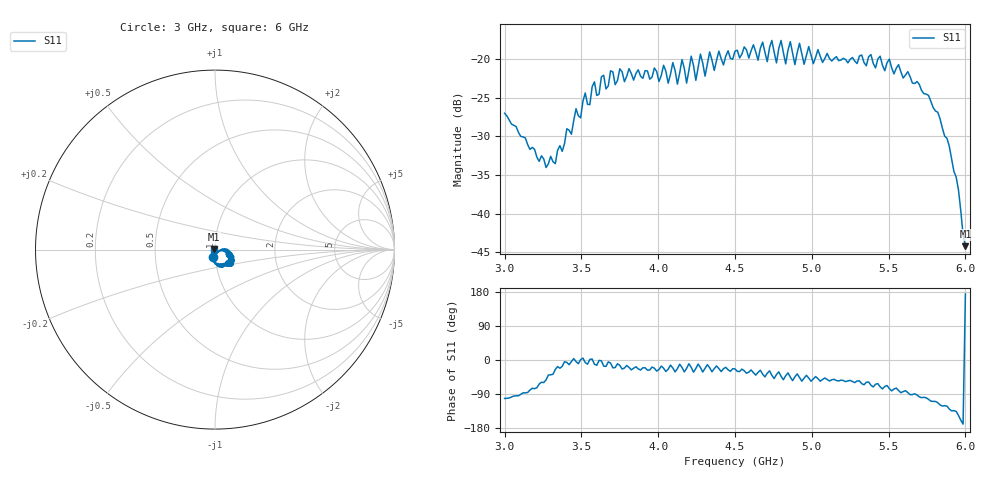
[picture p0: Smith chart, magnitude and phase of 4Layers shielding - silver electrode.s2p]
!  03/07/2025  16:02:48
! Ref Plane: 0.000 mm
# MHZ S MA R  50
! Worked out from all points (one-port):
!   201 points, 3 GHz to 6 GHz, reference 50 ohm
!   lowest |S11| = -44.2 dB at 6 GHz (marker M1), VSWR 1.01, Z = 49.4 + j0.0619 ohm
!   |S11| at or under -10 dB: start of sweep to end of sweep
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3000  0.0446 -101.5
3270  0.01987 -52.5
3375  0.02527 -16.7
3525  0.06031 -6.9
3555  0.0507 1.4
3585  0.0712 -11.3
3750  0.08648 -14.1
4005  0.07155 -25.4
4035  0.09118 -21.6
4065  0.06976 -24.2
4095  0.09481 -21.0
4125  0.06882 -22.9
4155  0.09917 -19.6
4185  0.06993 -22.0
4215  0.1044 -19.4
4245  0.07283 -22.4
4275  0.1077 -19.8
4305  0.07751 -22.3
4335  0.1112 -20.4
4365  0.08439 -22.8
4395  0.1125 -22.7
4500  0.1124 -23.6
4875  0.1088 -54.4
5250  0.09965 -53.9
5625  0.08282 -85.8
5880  0.0307 -121.7
5955  0.01422 -146.3
6000  0.006155 174.2
